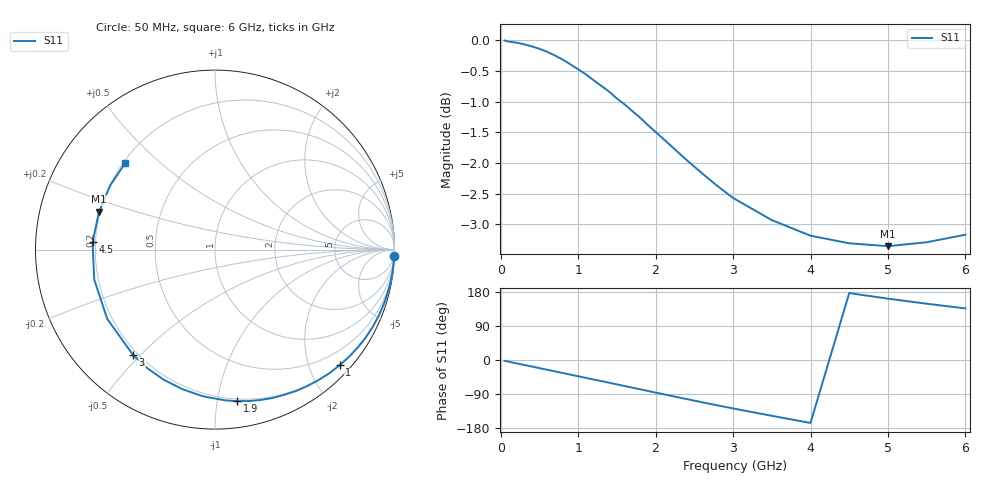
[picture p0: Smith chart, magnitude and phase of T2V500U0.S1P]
! SIEMENS Discrete & RF Semiconductors
! BAS70-04W
! Si Schottky Diode in SOT323
! VR = 0.5 V
! S-Parameters:  November  1997
# GHz  S  MA  R  50
!  f  S11
! GHz  MAG  ANG
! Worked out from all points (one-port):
!   34 points, 50 MHz to 6 GHz, reference 50 ohm
!   lowest |S11| = -3.4 dB at 5 GHz (marker M1), VSWR 5.24, Z = 9.77 + j7.67 ohm
!   |S11| at or under -10 dB: nowhere
!   S11 on the Smith chart (normalised r, x): 50 MHz: 0, -52; 1 GHz: 0.20, -2.53; 1.9 GHz: 0.18, -1.14; 3 GHz: 0.18, -0.48; 4.5 GHz: 0.19, +0.03; 6 GHz: 0.21, +0.39
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0.05  1 -2.2
0.2  0.9959 -8.7
0.3  0.9928 -13.0
0.4  0.9889 -17.2
0.5  0.9844 -21.5
0.6  0.9789 -25.8
0.7  0.9721 -30.0
0.8  0.9647 -34.3
1  0.9472 -42.9
1.1  0.9384 -47.2
1.2  0.928 -51.5
1.3  0.9182 -55.7
1.4  0.9083 -60.0
1.6  0.8869 -68.7
1.8  0.8651 -77.3
1.9  0.8531 -81.7
2  0.8422 -86.0
2.2  0.8204 -94.6
2.4  0.799 -103.0
2.6  0.7793 -111.5
2.8  0.7608 -119.7
3  0.7441 -127.8
3.5  0.7138 -147.3
4  0.6932 -166.1
4.5  0.6834 176.6
5  0.6797 161.9
5.5  0.6847 148.5
6  0.6945 136.2
